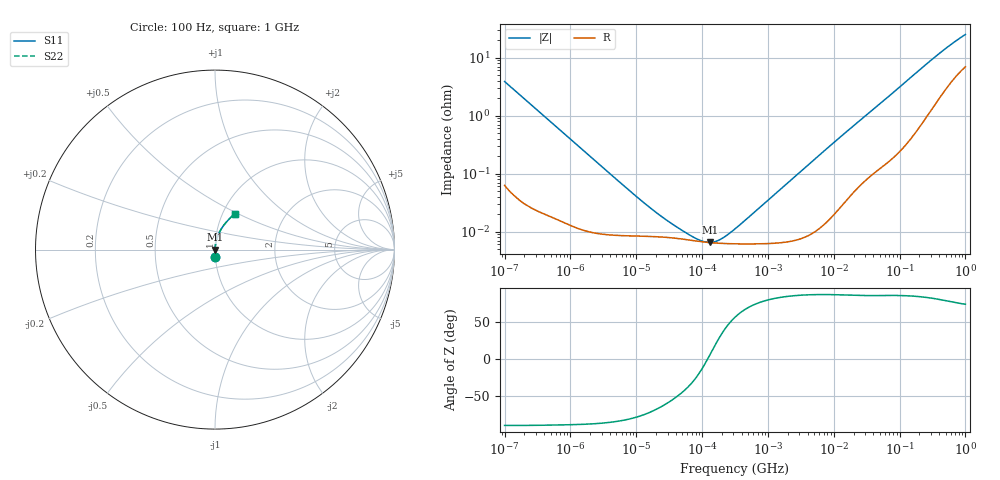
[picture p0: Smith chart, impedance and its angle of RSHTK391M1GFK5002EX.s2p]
! RSHTK391M1GFK5002EX  S-PARAMETER MODEL  (General Type)
! Model Generated by ELNA Corporation (http://www.ty-top.com)
! Version 1.0
! ELNA Control No. 201216
! Copyright (c) 2020 ELNA CO.,LTD. All Rights Reserved.
! Products Name : CONDUCTIVE POLYMER HYBRID ALUMINUM ELECTROLYTIC CAPACITORS
! Characteristics :
!  Capacitance  :  390uF  ,  Rated voltage  :  35V
!  Operating Temp. Range  :  -55 to +125 degC  ,  Endurance  :  4000hr at 125 degC
!  Dimension D  :  10mm  ,  Dimension L  :  12.5mm
! Frequency Range : 100Hz - 1GHz
! External Node Assignments :
!  1  o---| |---o  2
# MHz S RI R 50
!Freq[MHz].  S11 Real  S11 Imag  S21 Real  S21 Imag  S12 Real  S12 Imag  S22 Real  S22 Imag
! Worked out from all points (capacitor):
!   401 points, 100 Hz to 1 GHz, reference 50 ohm
!   read as one part in series: C = 411 uF near 108 Hz
!   lowest |Z| = 6.5 mohm at 130.3 kHz (marker M1)
!   series resonance near 121.1 kHz, so ESL is about 4.2 nH
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0.0001  0.00212 -0.0386  0.9979 0.0386  0.9979 0.0386  0.00212 -0.0386
0.000113  0.00171 -0.0343  0.9983 0.0343  0.9983 0.0343  0.00171 -0.0343
0.000285  0.000424 -0.0136  0.9996 0.0136  0.9996 0.0136  0.000424 -0.0136
0.001488  0.000115 -0.00265  0.9999 0.00265  0.9999 0.00265  0.000115 -0.00265
0.00912  8.42e-05 -0.000434  0.9999 0.000434  0.9999 0.000434  8.42e-05 -0.000434
0.014791  8.28e-05 -0.000268  0.9999 0.000268  0.9999 0.000268  8.28e-05 -0.000268
0.022131  8.12e-05 -0.000179  0.9999 0.000179  0.9999 0.000179  8.12e-05 -0.000179
0.038905  7.7e-05 -9.88e-05  0.9999 9.88e-05  0.9999 9.88e-05  7.7e-05 -9.88e-05
0.049545  7.45e-05 -7.41e-05  0.9999 7.41e-05  0.9999 7.41e-05  7.45e-05 -7.41e-05
0.053703  7.36e-05 -6.66e-05  0.9999 6.66e-05  0.9999 6.66e-05  7.36e-05 -6.66e-05
0.130317  6.47e-05 5.91e-06  0.9999 -5.91e-06  0.9999 -5.91e-06  6.47e-05 5.91e-06
0.258523  6.19e-05 6.91e-05  0.9999 -6.91e-05  0.9999 -6.91e-05  6.19e-05 6.91e-05
0.291743  6.17e-05 8.28e-05  0.9999 -8.28e-05  0.9999 -8.28e-05  6.17e-05 8.28e-05
0.316228  6.16e-05 9.27e-05  0.9999 -9.27e-05  0.9999 -9.27e-05  6.16e-05 9.27e-05
4.704354  9.54e-05 0.00162  0.9999 -0.00162  0.9999 -0.00162  9.54e-05 0.00162
14.53784  0.000339 0.00491  0.9997 -0.00491  0.9997 -0.00491  0.000339 0.00491
69.9842  0.00211 0.0218  0.9979 -0.0218  0.9979 -0.0218  0.00211 0.0218
176.8072  0.00801 0.0532  0.992 -0.0532  0.992 -0.0532  0.00801 0.0532
380.1894  0.0293 0.1057  0.9707 -0.1057  0.9707 -0.1057  0.0293 0.1057
668.3439  0.0685 0.1594  0.9315 -0.1594  0.9315 -0.1594  0.0685 0.1594
922.5714  0.1011 0.1922  0.8989 -0.1922  0.8989 -0.1922  0.1011 0.1922
1000  0.1101 0.2006  0.8899 -0.2006  0.8899 -0.2006  0.1101 0.2006
